(* Logix 5000 AddOnInstructionDefinition export HI1734_Faceplate_IT_AOI; software revision 30.00 *)

ADD_ON_INSTRUCTION HI1734_Faceplate_IT_AOI   (* revision 1.6, vendor Hardy Process Solutions *)
// For Integrated Technician data
VAR_IN_OUT
   Inp_hi1734 : HI:1734_WS:I:0; {required}
   Out_hi1734 : HI:1734_WS:O:0; {required}
END_VAR
VAR_INPUT
   IT_Status : DINT;   // Integrated Technician status indication
   pm_4990 : REAL;   // WT ch 0
   pm_4991 : REAL;   // Wt ch 1
   pm_4992 : REAL;   // WT ch 2
   pm_4993 : REAL;   // WT ch 3
   pm_4994 : REAL;   // WT ch 4
   pm_4995 : REAL;   // WT ch 5
   pm_4996 : REAL;   // WT ch 6
   pm_4997 : REAL;   // WT ch 7
   pm_49A0 : REAL;   // mv/v ch 0
   pm_49A1 : REAL;   // mv/v ch 1
   pm_49A2 : REAL;   // mv/v ch 2
   pm_49A3 : REAL;   // mv/v ch 3
   pm_49A8 : REAL;   // mv/v ref 1
   pm_49A4 : REAL;   // mv/v ch 4
   pm_49A5 : REAL;   // mv/v ch 5
   pm_49A6 : REAL;   // mv/v ch 6
   pm_49A7 : REAL;   // mv/v ch 7
   pm_49A9 : REAL;   // mv/v ref 2
   pm_49B0 : REAL;   // RAW VAR ch 0
   pm_49B1 : REAL;   // RAW VAR ch 1
   pm_49B2 : REAL;   // RAW VAR ch 2
   pm_49B3 : REAL;   // RAW VAR ch 3
   pm_49B8 : REAL;   // RAW VAR ref 1
   pm_49B4 : REAL;   // RAW VAR ch 4
   pm_49B5 : REAL;   // RAW VAR ch 5
   pm_49B6 : REAL;   // RAW VAR ch 6
   pm_49B7 : REAL;   // RAW VAR ch 7
   pm_49B9 : REAL;   // RAW VAR ref 2
   pm_49C0 : REAL;   // WAVERSAVER VAR ch 0
   pm_49C1 : REAL;   // WAVERSAVER VAR ch 1
   pm_49C2 : REAL;   // WAVERSAVER VAR ch 2
   pm_49C3 : REAL;   // WAVERSAVER VAR ch 3
   pm_49C8 : REAL;   // WAVERSAVER VAR ref 1
   pm_49C4 : REAL;   // WAVERSAVER VAR ch 4
   pm_49C5 : REAL;   // WAVERSAVER VAR ch 5
   pm_49C6 : REAL;   // WAVERSAVER VAR ch 6
   pm_49C7 : REAL;   // WAVERSAVER VAR ch 7
   pm_49C9 : REAL;   // WAVERSAVER VAR ref 2
   pm_49D0 : DINT;   // RAW VAR results ch 0
   pm_49D1 : DINT;   // RAW VAR results ch 1
   pm_49D2 : DINT;   // RAW VAR results ch 2
   pm_49D3 : DINT;   // RAW VAR results ch 3
   pm_49D8 : DINT;   // RAW VAR results ref 1
   pm_49D4 : DINT;   // RAW VAR results ch 4
   pm_49D5 : DINT;   // RAW VAR results ch 5
   pm_49D6 : DINT;   // RAW VAR results ch 6
   pm_49D7 : DINT;   // RAW VAR results ch 7
   pm_49D9 : DINT;   // RAW VAR results ref 2
   pm_49E0 : DINT;   // WAVERSAVER VAR results ch 0
   pm_49E1 : DINT;   // WAVERSAVER VAR results ch 1
   pm_49E2 : DINT;   // WAVERSAVER VAR results ch 2
   pm_49E3 : DINT;   // WAVERSAVER VAR results ch 3
   pm_49E8 : DINT;   // WAVERSAVER VAR results ref 1
   pm_49E4 : DINT;   // WAVERSAVER VAR results ch 4
   pm_49E5 : DINT;   // WAVERSAVER VAR results ch 5
   pm_49E6 : DINT;   // WAVERSAVER VAR results ch 6
   pm_49E7 : DINT;   // WAVERSAVER VAR results ch 7
   pm_49E9 : DINT;   // WAVERSAVER VAR results ref 2
   rd_rtz : INT;   // return to zero status
   pm_49F0 : DINT;   // RTZ ch 0
   pm_49F1 : DINT;   // RTZ ch 1
   pm_49F2 : DINT;   // RTZ ch 2
   pm_49F3 : DINT;   // RTZ ch 3
   pm_49F4 : DINT;   // RTZ ch 4
   pm_49F5 : DINT;   // RTZ ch 5
   pm_49F6 : DINT;   // RTZ ch 6
   pm_49F7 : DINT;   // RTZ ch 7
   pm_498C : DINT;   // RTZ combined
   IT_button : INT;   // IT cmd from faceplate
        .0   // IT cmd from faceplate
   pm_4881 : DINT;   // Number IT jboxes
   pm_4103 : DINT;   // Number C2 sensors
   pm_498D : DINT;   // num sensors jbox 1
   pm_498E : DINT;   // num sensors jbox 2
   IT_reduce_button : INT;   // IT reduced cmd from faceplate
        .0   // IT reduced cmd from faceplate
   IT_running_status : DINT;   // running/status indication
END_VAR
VAR
   rd_IT_wt : INT; {access None}   // Trigger to check weights
   rd_mVV : INT; {access None}   // trigger to read mv/v
   rd_raw_var : INT; {access None}   // trigger to read raw variation
   rd_ws_var : INT; {access None}   // trigger to read WAVERSAVER variation
   rd_raw_rst : INT; {access None}   // trigger to read raw variation results
   rd_ws_rst : INT; {access None}   // trigger to read WAVERSAVER results
   wr_jbox_2 : BOOL; {access None}   // Process control bit
   IT_request : INT; {access None}   // type 1=standard 2=reduced
   IT_cmd : INT;   // trigger to run IT test
   type_IT_cmd : BOOL; {access None}   // process control bit
   c2_search : BOOL; {access None}   // process control bit
   rd_C2_devices : BOOL; {access None}   // trigger to check for devices
   jbox_check : BOOL; {access None}   // j-box check process bit
   one_jbox : BOOL; {access None}   // One IT j-box found indication
   two_jbox : BOOL; {access None}   // two IT j-box indication
   run_IT_test : BOOL; {access None}   // Process control bit
   cmd_IT : DINT; {access None}   // holding register for command to be run
   IT_complete : BOOL; {access None}   // process status bit
   IT_failed : BOOL; {access None}   // process status bit
   start_timer100 : BOOL; {access None}   // process control bit
   delay100 : TIMER := (PRE := 500); {access None}   // delay to allow process to complete
   start_timer101 : BOOL; {access None}   // process control bit
   delay101 : TIMER := (PRE := 200); {access None}   // delay to allow process to complete
   start_timer102 : BOOL; {access None}   // process control bit
   delay102 : TIMER := (PRE := 200); {access None}   // delay to allow process to complete
   start_timer103 : BOOL; {access None}   // process control bit
   delay103 : TIMER := (PRE := 200); {access None}   // delay to allow process to complete
   start_timer104 : BOOL; {access None}   // process control bit
   delay104 : TIMER := (PRE := 200); {access None}   // delay to allow process to complete
   start_timer105 : BOOL; {access None}   // process control bit
   delay105 : TIMER := (PRE := 200); {access None}   // delay to allow process to complete
   start_timer106 : BOOL; {access None}   // process control bit
   delay106 : TIMER := (PRE := 200); {access None}   // delay to allow process to complete
   start_timer107 : BOOL; {access None}   // process control bit
   delay107 : TIMER := (PRE := 200); {access None}   // delay to allow process to complete
   start_timer108 : BOOL; {access None}   // process control bit
   delay108 : TIMER := (PRE := 200); {access None}   // delay to allow process to complete
   start_timer109 : BOOL; {access None}   // process control bit
   delay109 : TIMER := (PRE := 200); {access None}   // delay to allow process to complete
   start_timer110 : BOOL; {access None}   // process control bit
   delay110 : TIMER := (PRE := 200); {access None}   // delay to allow process to complete
   start_timer111 : BOOL; {access None}   // process control bit
   delay111 : TIMER := (PRE := 200); {access None}   // delay to allow process to complete
   start_timer112 : BOOL; {access None}   // process control bit
   delay112 : TIMER := (PRE := 200); {access None}   // delay to allow process to complete
   start_timer113 : BOOL; {access None}   // process control bit
   delay113 : TIMER := (PRE := 200); {access None}   // delay to allow process to complete
   start_timer114 : BOOL; {access None}   // process control bit
   delay114 : TIMER := (PRE := 200); {access None}   // delay to allow process to complete
   start_timer115 : BOOL; {access None}   // process control bit
   delay115 : TIMER := (PRE := 200); {access None}   // delay to allow process to complete
   start_timer116 : BOOL; {access None}   // process control bit
   delay116 : TIMER := (PRE := 200); {access None}   // delay to allow process to complete
   start_timer117 : BOOL; {access None}   // process control bit
   delay117 : TIMER := (PRE := 200); {access None}   // delay to allow process to complete
   start_timer118 : BOOL; {access None}   // process control bit
   start_timer119 : BOOL; {access None}   // process control bit
   delay118 : TIMER := (PRE := 200); {access None}   // delay to allow process to complete
   delay119 : TIMER := (PRE := 200); {access None}   // delay to allow process to complete
   start_timer120 : BOOL; {access None}   // process control bit
   delay120 : TIMER := (PRE := 200); {access None}   // delay to allow process to complete
   start_timer121 : BOOL; {access None}   // process control bit
   delay121 : TIMER := (PRE := 200); {access None}   // delay to allow process to complete
   start_timer122 : BOOL; {access None}   // process control bit
   delay122 : TIMER := (PRE := 200); {access None}   // delay to allow process to complete
   start_timer123 : BOOL; {access None}   // process control bit
   delay123 : TIMER := (PRE := 200); {access None}   // delay to allow process to complete
   start_timer124 : BOOL; {access None}   // process control bit
   delay124 : TIMER := (PRE := 200); {access None}   // delay to allow process to complete
   start_timer125 : BOOL; {access None}   // process control bit
   delay125 : TIMER := (PRE := 200); {access None}   // delay to allow process to complete
   start_timer126 : BOOL; {access None}   // process control bit
   delay126 : TIMER := (PRE := 200); {access None}   // delay to allow process to complete
   start_timer127 : BOOL; {access None}   // process control bit
   delay127 : TIMER := (PRE := 200); {access None}   // delay to allow process to complete
   start_timer128 : BOOL; {access None}   // process control bit
   delay128 : TIMER := (PRE := 200); {access None}   // delay to allow process to complete
   start_timer129 : BOOL; {access None}   // process control bit
   delay129 : TIMER := (PRE := 200); {access None}   // delay to allow process to complete
   start_timer130 : BOOL; {access None}   // process control bit
   delay130 : TIMER := (PRE := 200); {access None}   // delay to allow process to complete
   start_timer131 : BOOL; {access None}   // process control bit
   delay131 : TIMER := (PRE := 200); {access None}   // delay to allow process to complete
   start_timer132 : BOOL; {access None}   // process control bit
   delay132 : TIMER := (PRE := 200); {access None}   // delay to allow process to complete
   start_timer133 : BOOL; {access None}   // process control bit
   delay133 : TIMER := (PRE := 200); {access None}   // delay to allow process to complete
   start_timer134 : BOOL; {access None}   // process control bit
   writ_box1_lc_cnt : BOOL; {access None}   // Process control bit
   delay134 : TIMER := (PRE := 200); {access None}   // delay to allow process to complete
   writ_box2_lc_cnt : BOOL; {access None}   // Process control bit
   start_timer135 : BOOL; {access None}   // process control bit
   delay135 : TIMER := (PRE := 200); {access None}   // delay to allow process to complete
   run_C2_search : BOOL; {access None}   // Process control bit
   c2_dev_notmatch : BOOL; {access None}   // status indication bit
   total_sensors : DINT; {access None}   // total sensors indication
   clear_status : BOOL; {access None}   // process control bit
   delay138 : TIMER := (PRE := 5000); {access None}   // delay to allow process to complete
   start_timer139 : BOOL; {access None}   // process control bit
   delay139 : TIMER := (PRE := 200); {access None}   // delay to allow process to complete
   start_timer141 : BOOL; {access None}   // process control bit
   delay142 : TIMER := (PRE := 2000); {access None}   // delay to allow process to complete
   no_it_jbox : BOOL; {access None}   // no IT j-box indication
   rd_jbox_2_too : BOOL; {access None}   // Process control bit
END_VAR

ROUTINE Logic   (* ladder *)
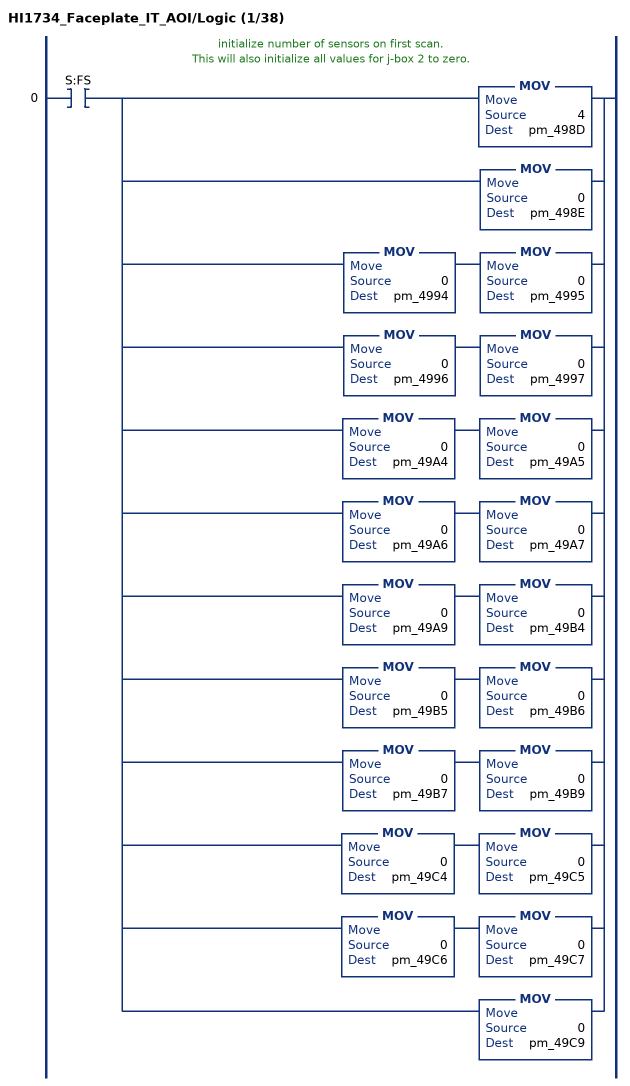
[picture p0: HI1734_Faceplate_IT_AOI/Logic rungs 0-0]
   // initialize number of sensors on first scan.
   // This will also initialize all values for j-box 2 to zero.
   0: XIC(S:FS)[MOV(4,pm_498D) ,MOV(0,pm_498E) ,MOV(0,pm_4994) MOV(0,pm_4995) ,MOV(0,pm_4996) MOV(0,pm_4997) ,MOV(0,pm_49A4) MOV(0,pm_49A5) ,MOV(0,pm_49A6) MOV(0,pm_49A7) ,MOV(0,pm_49A9) MOV(0,pm_49B4) ,MOV(0,pm_49B5) MOV(0,pm_49B6) ,MOV(0,pm_49B7) MOV(0,pm_49B9) ,MOV(0,pm_49C4) MOV(0,pm_49C5) ,MOV(0,pm_49C6) MOV(0,pm_49C7) ,MOV(0,pm_49C9) ];
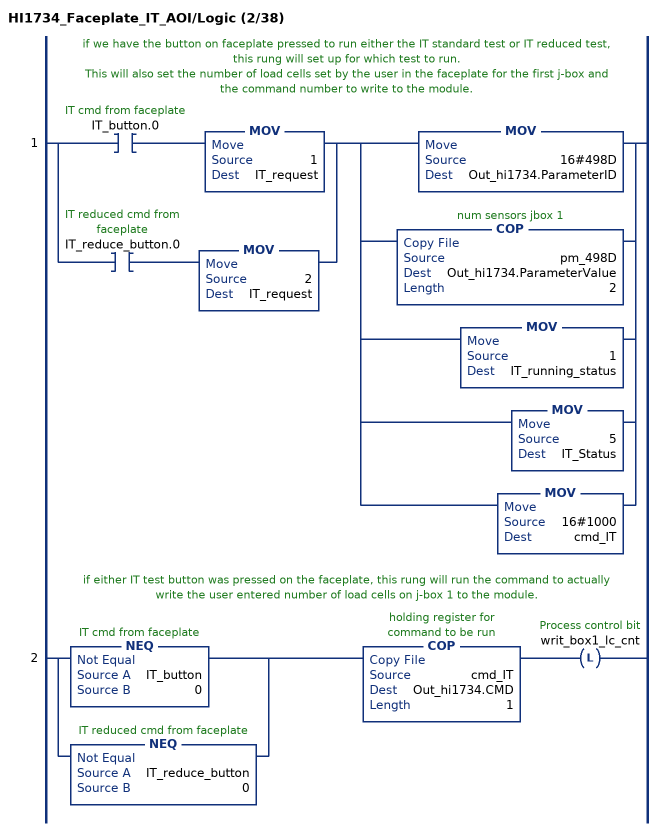
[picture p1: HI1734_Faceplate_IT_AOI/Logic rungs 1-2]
   // if we have the button on faceplate pressed to run either the IT standard test or IT reduced test, this rung will set up for which test to run.
   // This will also set the number of load cells set by the user in the faceplate for the first j-box and the command number to write to the module.
   1: [XIC(IT_button.0) MOV(1,IT_request) ,XIC(IT_reduce_button.0) MOV(2,IT_request) ][MOV(16#498D,Out_hi1734.ParameterID) ,COP(pm_498D,Out_hi1734.ParameterValue,2) ,MOV(1,IT_running_status) ,MOV(5,IT_Status) ,MOV(16#1000,cmd_IT) ];
   // if either IT test button was pressed on the faceplate, this rung will run the command to actually write the user entered number of load cells on j-box 1 to the module.
   2: [NEQ(IT_button,0) ,NEQ(IT_reduce_button,0) ]COP(cmd_IT,Out_hi1734.CMD,1)OTL(writ_box1_lc_cnt);
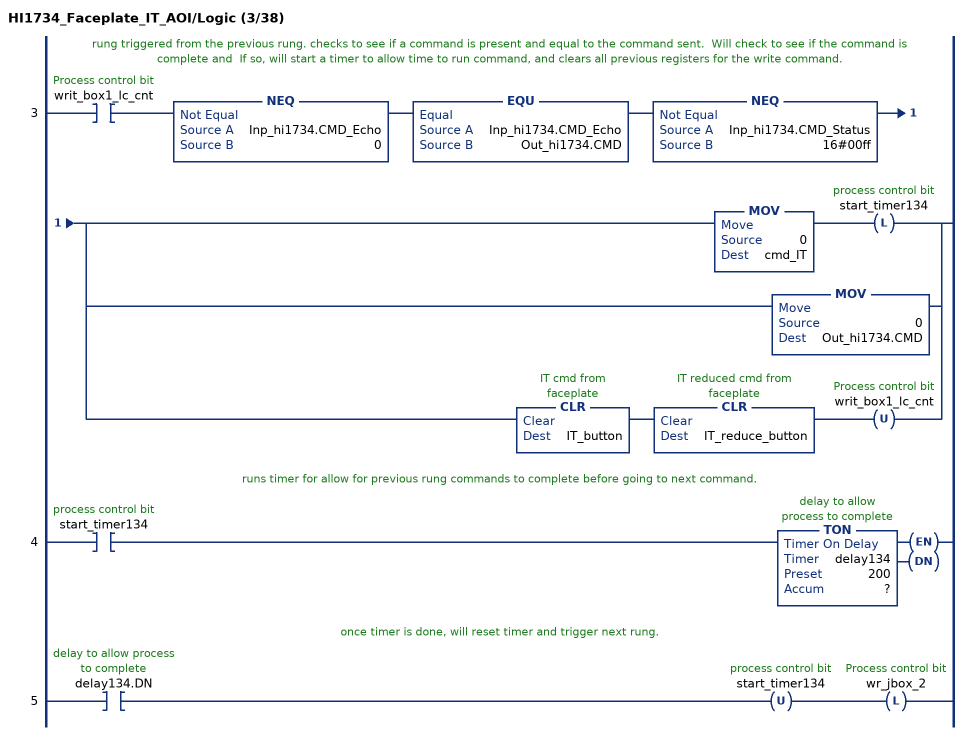
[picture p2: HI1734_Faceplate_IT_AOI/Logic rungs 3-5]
   // rung triggered from the previous rung. checks to see if a command is present and equal to the command sent.  Will check to see if the command is complete and  If so, will start a timer to allow time to run command, and clears all previous registers for the write command.
   3: XIC(writ_box1_lc_cnt)NEQ(Inp_hi1734.CMD_Echo,0)EQU(Inp_hi1734.CMD_Echo,Out_hi1734.CMD)NEQ(Inp_hi1734.CMD_Status,16#00ff)[MOV(0,cmd_IT) OTL(start_timer134) ,MOV(0,Out_hi1734.CMD) ,CLR(IT_button) CLR(IT_reduce_button) OTU(writ_box1_lc_cnt) ];
   // runs timer for allow for previous rung commands to complete before going to next command.
   4: XIC(start_timer134)TON(delay134,?,?);
   // once timer is done, will reset timer and trigger next rung.
   5: XIC(delay134.DN)OTU(start_timer134)OTL(wr_jbox_2);
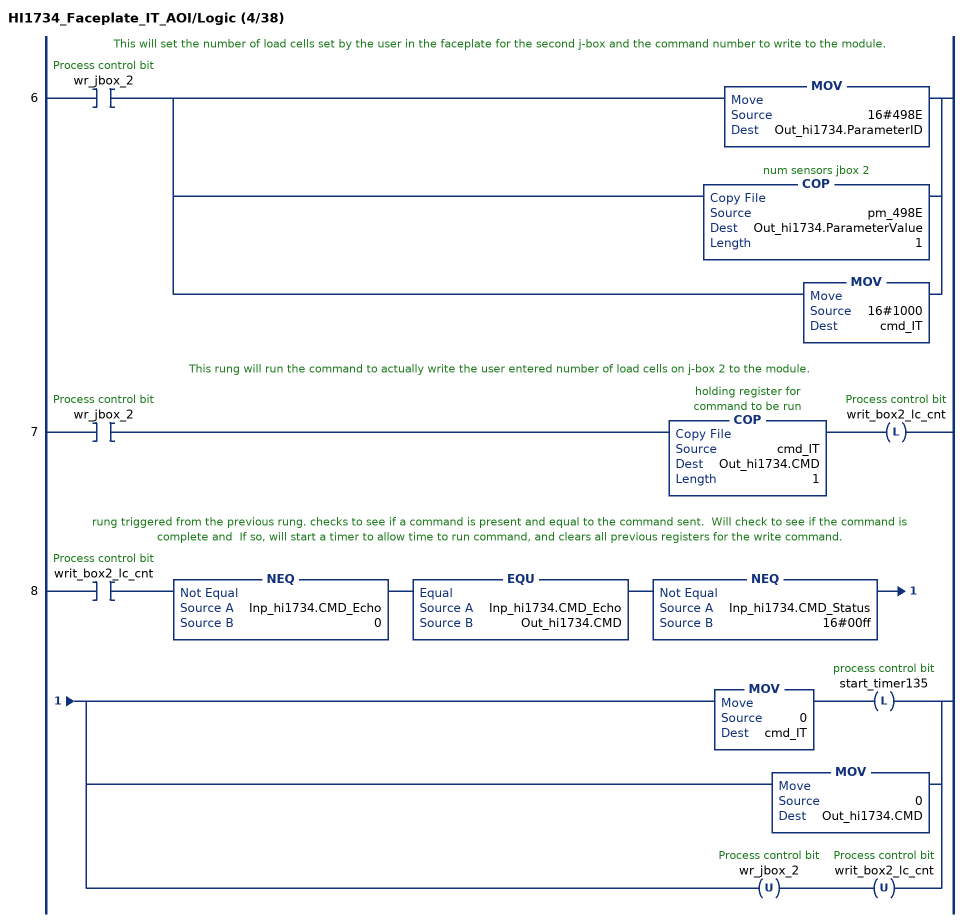
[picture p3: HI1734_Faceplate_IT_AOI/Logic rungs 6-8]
   // This will set the number of load cells set by the user in the faceplate for the second j-box and the command number to write to the module.
   6: XIC(wr_jbox_2)[MOV(16#498E,Out_hi1734.ParameterID) ,COP(pm_498E,Out_hi1734.ParameterValue,1) ,MOV(16#1000,cmd_IT) ];
   // This rung will run the command to actually write the user entered number of load cells on j-box 2 to the module.
   7: XIC(wr_jbox_2)COP(cmd_IT,Out_hi1734.CMD,1)OTL(writ_box2_lc_cnt);
   // rung triggered from the previous rung. checks to see if a command is present and equal to the command sent.  Will check to see if the command is complete and  If so, will start a timer to allow time to run command, and clears all previous registers for the write command.
   8: XIC(writ_box2_lc_cnt)NEQ(Inp_hi1734.CMD_Echo,0)EQU(Inp_hi1734.CMD_Echo,Out_hi1734.CMD)NEQ(Inp_hi1734.CMD_Status,16#00ff)[MOV(0,cmd_IT) OTL(start_timer135) ,MOV(0,Out_hi1734.CMD) ,OTU(wr_jbox_2) OTU(writ_box2_lc_cnt) ];
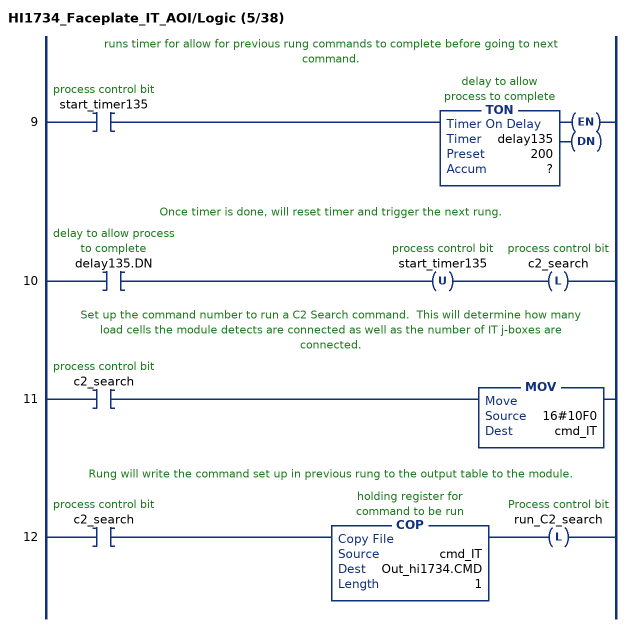
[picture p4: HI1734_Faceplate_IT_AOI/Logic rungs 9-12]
   // runs timer for allow for previous rung commands to complete before going to next command.
   9: XIC(start_timer135)TON(delay135,?,?);
   // Once timer is done, will reset timer and trigger the next rung.
   10: XIC(delay135.DN)OTU(start_timer135)OTL(c2_search);
   // Set up the command number to run a C2 Search command.  This will determine how many load cells the module detects are connected as well as the number of IT j-boxes are connected.
   11: XIC(c2_search)MOV(16#10F0,cmd_IT);
   // Rung will write the command set up in previous rung to the output table to the module.
   12: XIC(c2_search)COP(cmd_IT,Out_hi1734.CMD,1)OTL(run_C2_search);
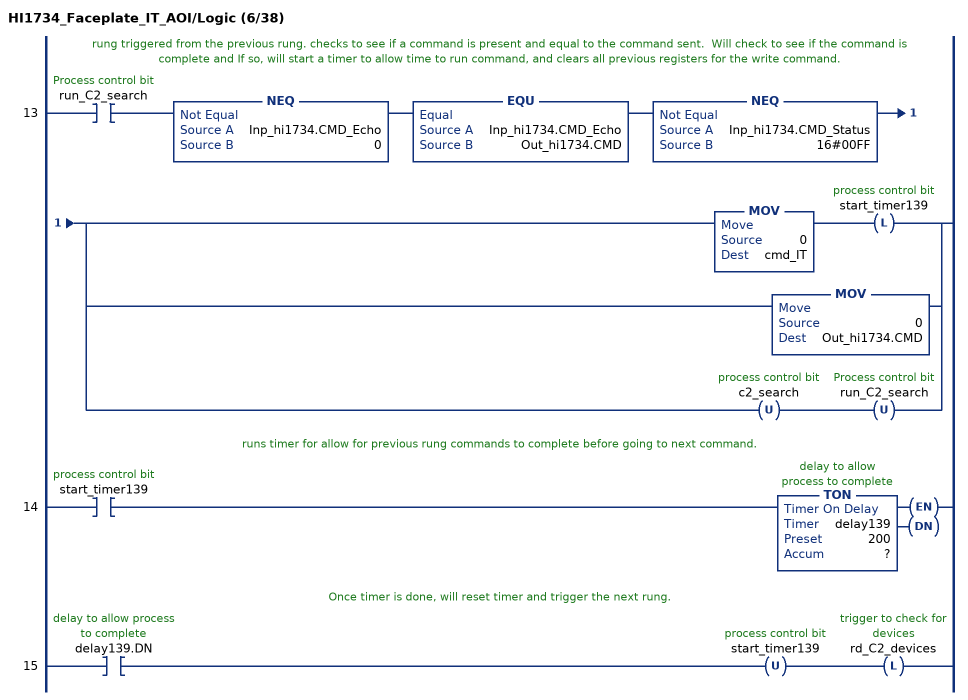
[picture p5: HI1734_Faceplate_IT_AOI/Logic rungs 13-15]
   // rung triggered from the previous rung. checks to see if a command is present and equal to the command sent.  Will check to see if the command is complete and If so, will start a timer to allow time to run command, and clears all previous registers for the write command.
   13: XIC(run_C2_search)NEQ(Inp_hi1734.CMD_Echo,0)EQU(Inp_hi1734.CMD_Echo,Out_hi1734.CMD)NEQ(Inp_hi1734.CMD_Status,16#00FF)[MOV(0,cmd_IT) OTL(start_timer139) ,MOV(0,Out_hi1734.CMD) ,OTU(c2_search) OTU(run_C2_search) ];
   // runs timer for allow for previous rung commands to complete before going to next command.
   14: XIC(start_timer139)TON(delay139,?,?);
   // Once timer is done, will reset timer and trigger the next rung.
   15: XIC(delay139.DN)OTU(start_timer139)OTL(rd_C2_devices);
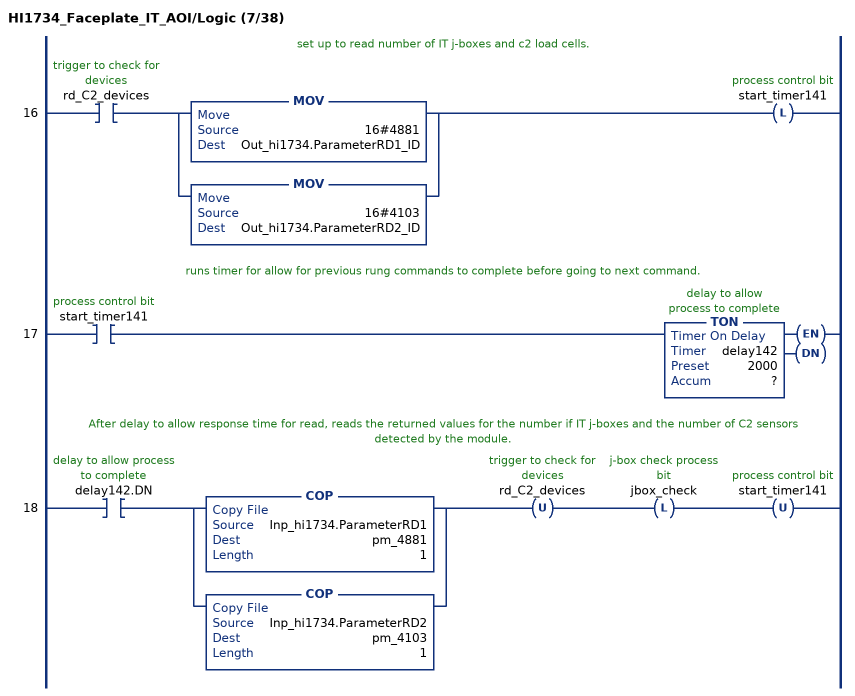
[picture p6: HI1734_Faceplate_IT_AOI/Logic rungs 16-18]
   // set up to read number of IT j-boxes and c2 load cells.
   16: XIC(rd_C2_devices)[MOV(16#4881,Out_hi1734.ParameterRD1_ID) ,MOV(16#4103,Out_hi1734.ParameterRD2_ID) ]OTL(start_timer141);
   // runs timer for allow for previous rung commands to complete before going to next command.
   17: XIC(start_timer141)TON(delay142,?,?);
   // After delay to allow response time for read, reads the returned values for the number if IT j-boxes and the number of C2 sensors detected by the module.
   18: XIC(delay142.DN)[COP(Inp_hi1734.ParameterRD1,pm_4881,1) ,COP(Inp_hi1734.ParameterRD2,pm_4103,1) ]OTU(rd_C2_devices)OTL(jbox_check)OTU(start_timer141);
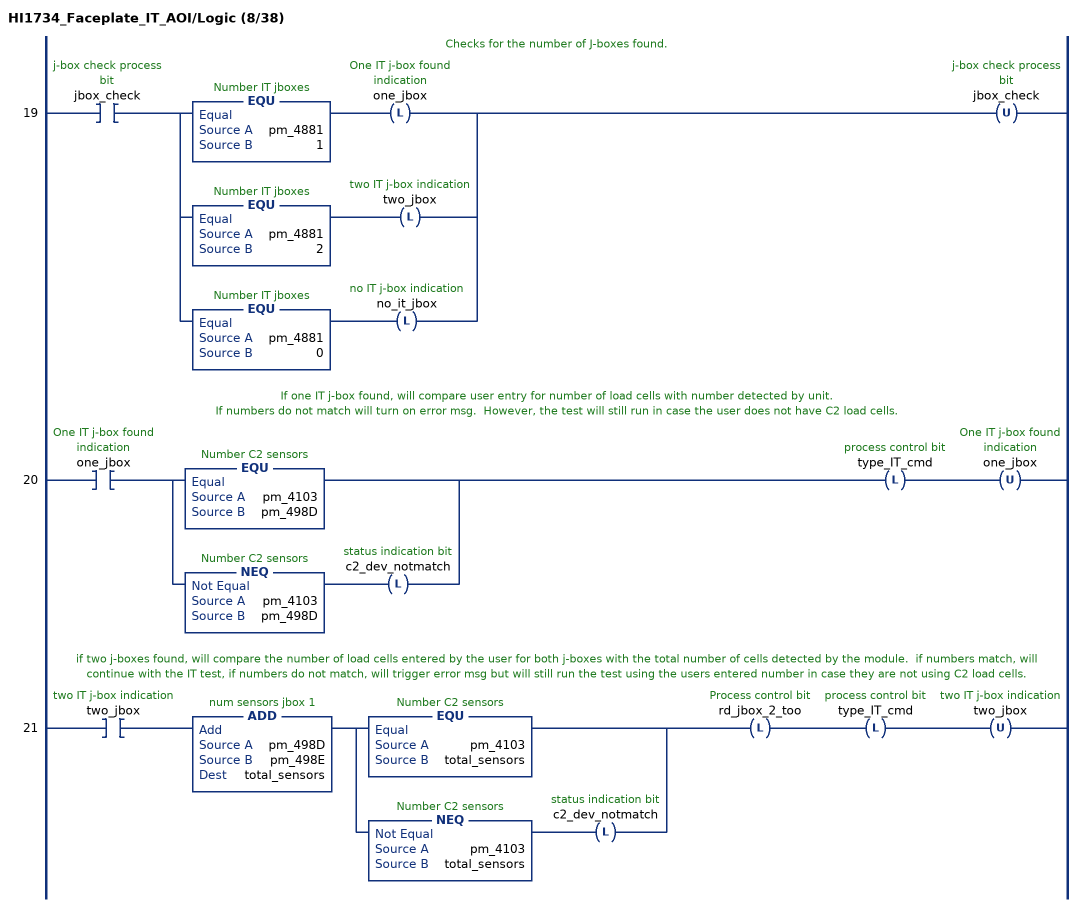
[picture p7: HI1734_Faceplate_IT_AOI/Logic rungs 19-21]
   // Checks for the number of J-boxes found.
   19: XIC(jbox_check)[EQU(pm_4881,1) OTL(one_jbox) ,EQU(pm_4881,2) OTL(two_jbox) ,EQU(pm_4881,0) OTL(no_it_jbox) ]OTU(jbox_check);
   // If one IT j-box found, will compare user entry for number of load cells with number detected by unit.
   // If numbers do not match will turn on error msg.  However, the test will still run in case the user does not have C2 load cells.
   20: XIC(one_jbox)[EQU(pm_4103,pm_498D) ,NEQ(pm_4103,pm_498D) OTL(c2_dev_notmatch) ]OTL(type_IT_cmd)OTU(one_jbox);
   // if two j-boxes found, will compare the number of load cells entered by the user for both j-boxes with the total number of cells detected by the module.  if numbers match, will continue with the IT test, if numbers do not match, will trigger error msg but will still run the test using the users entered number in case they are not using C2 load cells.
   21: XIC(two_jbox)ADD(pm_498D,pm_498E,total_sensors)[EQU(pm_4103,total_sensors) ,NEQ(pm_4103,total_sensors) OTL(c2_dev_notmatch) ]OTL(rd_jbox_2_too)OTL(type_IT_cmd)OTU(two_jbox);
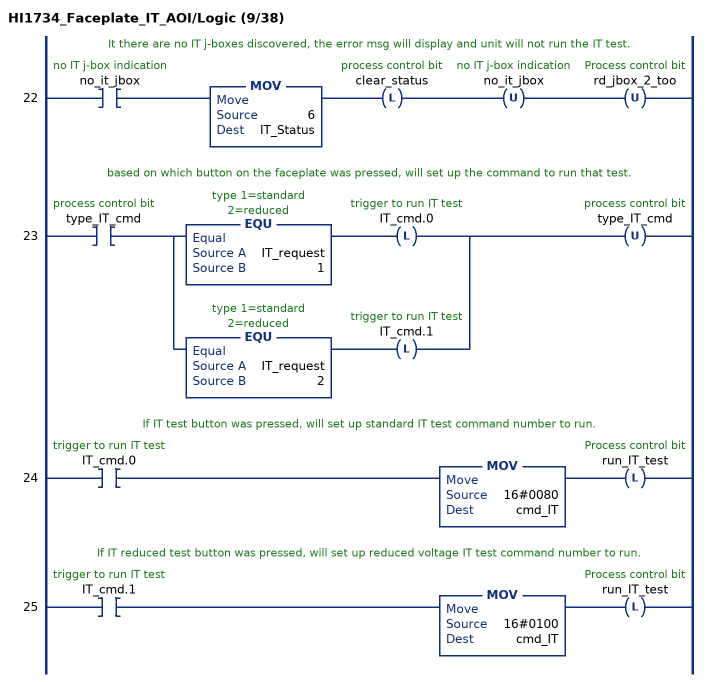
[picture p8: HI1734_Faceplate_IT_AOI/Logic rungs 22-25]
   // It there are no IT j-boxes discovered, the error msg will display and unit will not run the IT test.
   22: XIC(no_it_jbox)MOV(6,IT_Status)OTL(clear_status)OTU(no_it_jbox)OTU(rd_jbox_2_too);
   // based on which button on the faceplate was pressed, will set up the command to run that test.
   23: XIC(type_IT_cmd)[EQU(IT_request,1) OTL(IT_cmd.0) ,EQU(IT_request,2) OTL(IT_cmd.1) ]OTU(type_IT_cmd);
   // If IT test button was pressed, will set up standard IT test command number to run.
   24: XIC(IT_cmd.0)MOV(16#0080,cmd_IT)OTL(run_IT_test);
   // If IT reduced test button was pressed, will set up reduced voltage IT test command number to run.
   25: XIC(IT_cmd.1)MOV(16#0100,cmd_IT)OTL(run_IT_test);
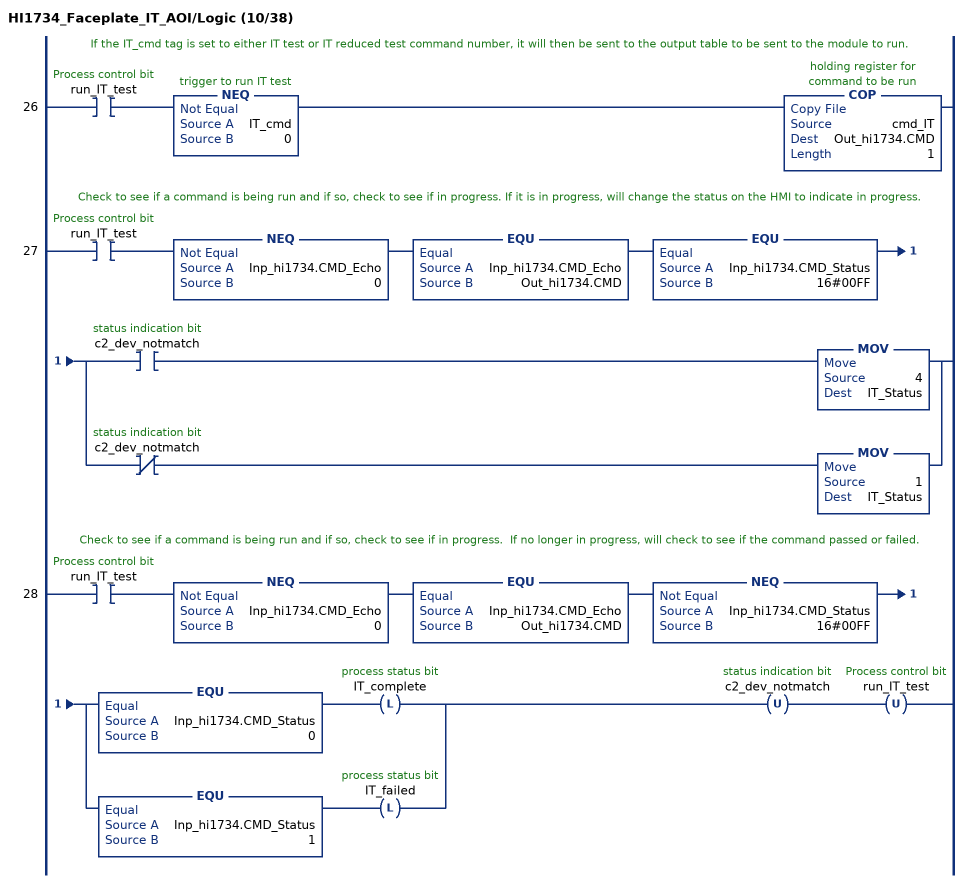
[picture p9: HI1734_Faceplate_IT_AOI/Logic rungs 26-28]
   // If the IT_cmd tag is set to either IT test or IT reduced test command number, it will then be sent to the output table to be sent to the module to run.
   26: XIC(run_IT_test)NEQ(IT_cmd,0)COP(cmd_IT,Out_hi1734.CMD,1);
   // Check to see if a command is being run and if so, check to see if in progress. If it is in progress, will change the status on the HMI to indicate in progress.
   27: XIC(run_IT_test)NEQ(Inp_hi1734.CMD_Echo,0)EQU(Inp_hi1734.CMD_Echo,Out_hi1734.CMD)EQU(Inp_hi1734.CMD_Status,16#00FF)[XIC(c2_dev_notmatch) MOV(4,IT_Status) ,XIO(c2_dev_notmatch) MOV(1,IT_Status) ];
   // Check to see if a command is being run and if so, check to see if in progress.  If no longer in progress, will check to see if the command passed or failed.
   28: XIC(run_IT_test)NEQ(Inp_hi1734.CMD_Echo,0)EQU(Inp_hi1734.CMD_Echo,Out_hi1734.CMD)NEQ(Inp_hi1734.CMD_Status,16#00FF)[EQU(Inp_hi1734.CMD_Status,0) OTL(IT_complete) ,EQU(Inp_hi1734.CMD_Status,1) OTL(IT_failed) ]OTU(c2_dev_notmatch)OTU(run_IT_test);
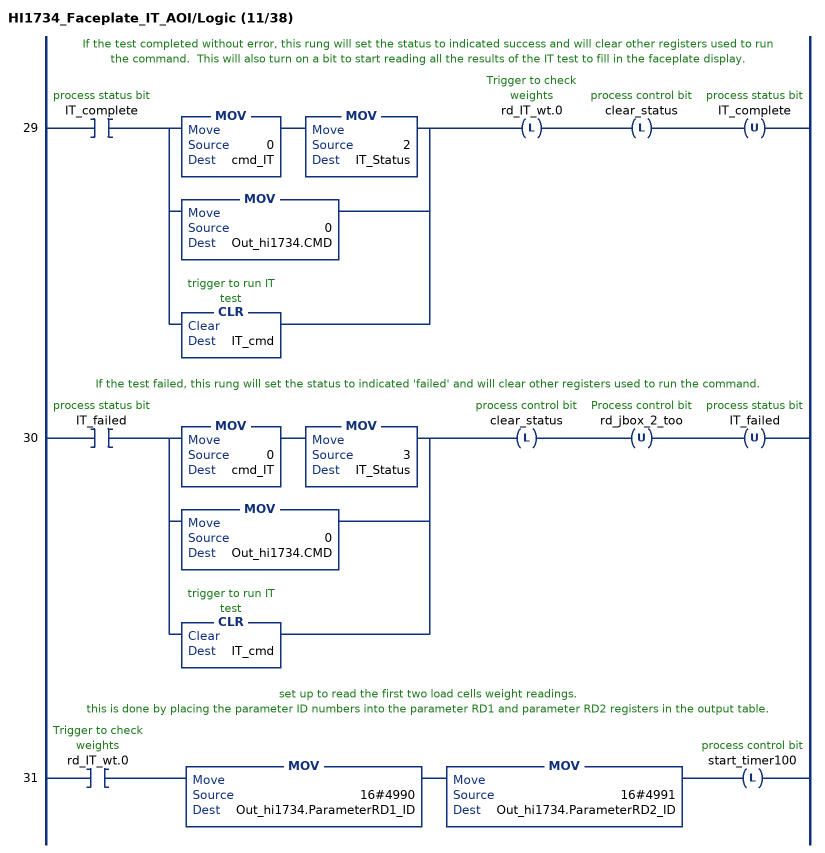
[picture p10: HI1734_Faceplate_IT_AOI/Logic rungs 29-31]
   // If the test completed without error, this rung will set the status to indicated success and will clear other registers used to run the command.  This will also turn on a bit to start reading all the results of the IT test to fill in the faceplate display.
   29: XIC(IT_complete)[MOV(0,cmd_IT) MOV(2,IT_Status) ,MOV(0,Out_hi1734.CMD) ,CLR(IT_cmd) ]OTL(rd_IT_wt.0)OTL(clear_status)OTU(IT_complete);
   // If the test failed, this rung will set the status to indicated 'failed' and will clear other registers used to run the command.
   30: XIC(IT_failed)[MOV(0,cmd_IT) MOV(3,IT_Status) ,MOV(0,Out_hi1734.CMD) ,CLR(IT_cmd) ]OTL(clear_status)OTU(rd_jbox_2_too)OTU(IT_failed);
   // set up to read the first two load cells weight readings.
   // this is done by placing the parameter ID numbers into the parameter RD1 and parameter RD2 registers in the output table.
   31: XIC(rd_IT_wt.0)MOV(16#4990,Out_hi1734.ParameterRD1_ID)MOV(16#4991,Out_hi1734.ParameterRD2_ID)OTL(start_timer100);
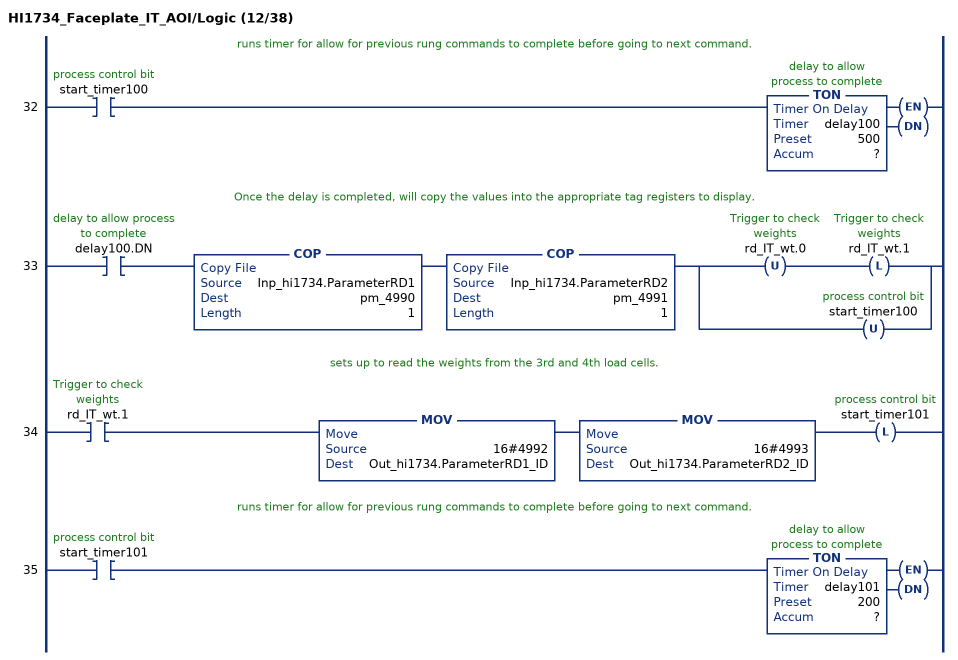
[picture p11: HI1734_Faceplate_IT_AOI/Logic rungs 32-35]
   // runs timer for allow for previous rung commands to complete before going to next command.
   32: XIC(start_timer100)TON(delay100,?,?);
   // Once the delay is completed, will copy the values into the appropriate tag registers to display.
   33: XIC(delay100.DN)COP(Inp_hi1734.ParameterRD1,pm_4990,1)COP(Inp_hi1734.ParameterRD2,pm_4991,1)[OTU(rd_IT_wt.0) OTL(rd_IT_wt.1) ,OTU(start_timer100) ];
   // sets up to read the weights from the 3rd and 4th load cells.
   34: XIC(rd_IT_wt.1)MOV(16#4992,Out_hi1734.ParameterRD1_ID)MOV(16#4993,Out_hi1734.ParameterRD2_ID)OTL(start_timer101);
   // runs timer for allow for previous rung commands to complete before going to next command.
   35: XIC(start_timer101)TON(delay101,?,?);
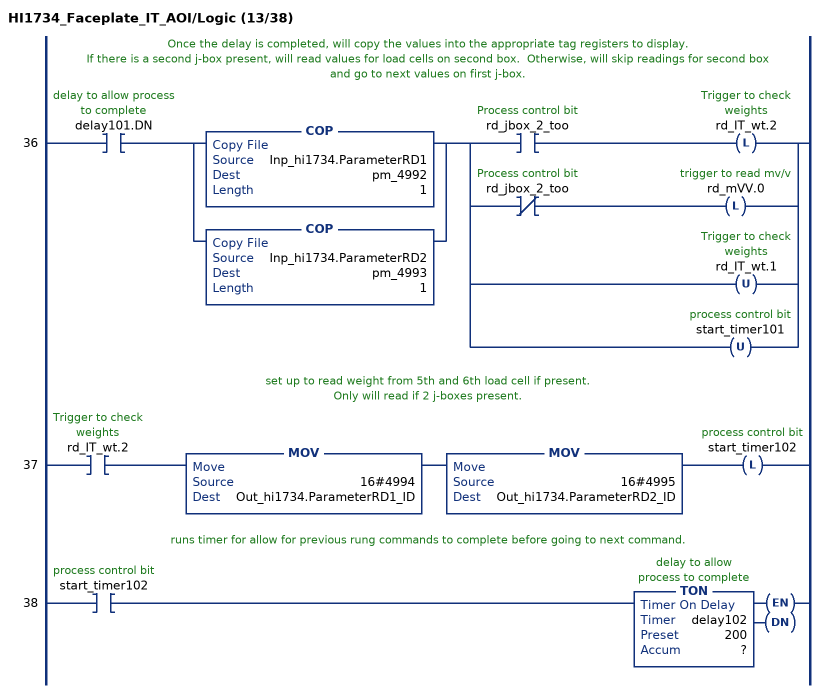
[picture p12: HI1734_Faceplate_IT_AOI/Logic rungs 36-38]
   // Once the delay is completed, will copy the values into the appropriate tag registers to display.
   // If there is a second j-box present, will read values for load cells on second box.  Otherwise, will skip readings for second box and go to next values on first j-box.
   36: XIC(delay101.DN)[COP(Inp_hi1734.ParameterRD1,pm_4992,1) ,COP(Inp_hi1734.ParameterRD2,pm_4993,1) ][XIC(rd_jbox_2_too) OTL(rd_IT_wt.2) ,XIO(rd_jbox_2_too) OTL(rd_mVV.0) ,OTU(rd_IT_wt.1) ,OTU(start_timer101) ];
   // set up to read weight from 5th and 6th load cell if present.
   // Only will read if 2 j-boxes present.
   37: XIC(rd_IT_wt.2)MOV(16#4994,Out_hi1734.ParameterRD1_ID)MOV(16#4995,Out_hi1734.ParameterRD2_ID)OTL(start_timer102);
   // runs timer for allow for previous rung commands to complete before going to next command.
   38: XIC(start_timer102)TON(delay102,?,?);
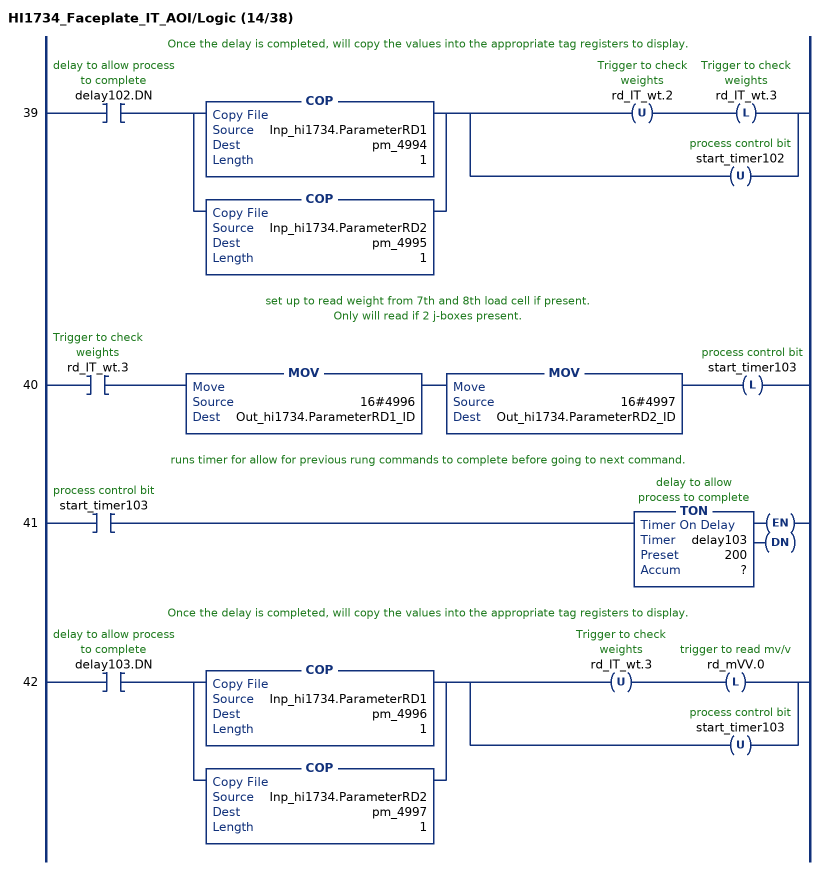
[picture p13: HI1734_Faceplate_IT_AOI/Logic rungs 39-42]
   // Once the delay is completed, will copy the values into the appropriate tag registers to display.
   39: XIC(delay102.DN)[COP(Inp_hi1734.ParameterRD1,pm_4994,1) ,COP(Inp_hi1734.ParameterRD2,pm_4995,1) ][OTU(rd_IT_wt.2) OTL(rd_IT_wt.3) ,OTU(start_timer102) ];
   // set up to read weight from 7th and 8th load cell if present.
   // Only will read if 2 j-boxes present.
   40: XIC(rd_IT_wt.3)MOV(16#4996,Out_hi1734.ParameterRD1_ID)MOV(16#4997,Out_hi1734.ParameterRD2_ID)OTL(start_timer103);
   // runs timer for allow for previous rung commands to complete before going to next command.
   41: XIC(start_timer103)TON(delay103,?,?);
   // Once the delay is completed, will copy the values into the appropriate tag registers to display.
   42: XIC(delay103.DN)[COP(Inp_hi1734.ParameterRD1,pm_4996,1) ,COP(Inp_hi1734.ParameterRD2,pm_4997,1) ][OTU(rd_IT_wt.3) OTL(rd_mVV.0) ,OTU(start_timer103) ];
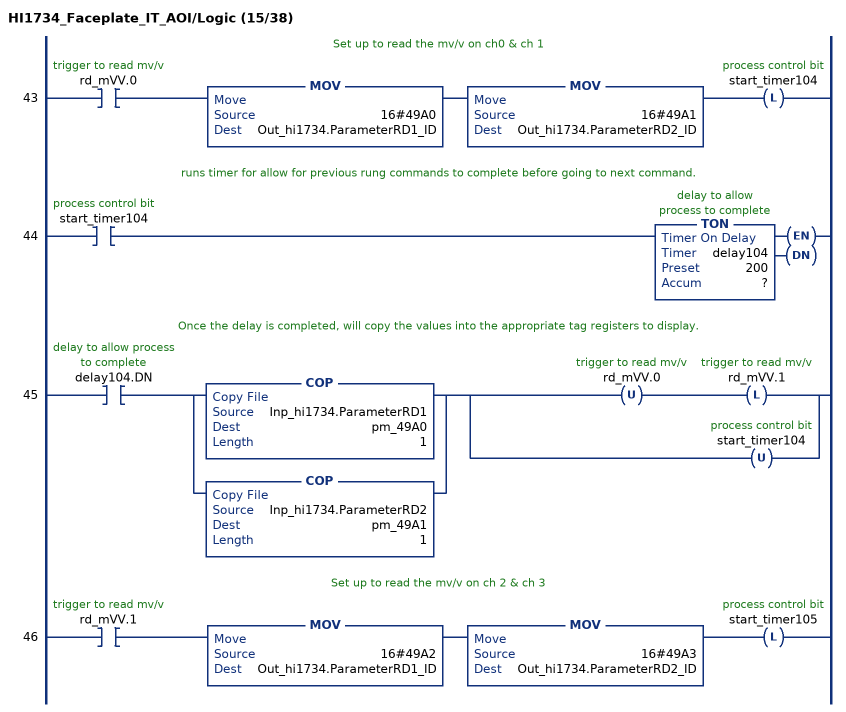
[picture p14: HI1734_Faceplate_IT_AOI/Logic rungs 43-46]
   // Set up to read the mv/v on ch0 & ch 1
   43: XIC(rd_mVV.0)MOV(16#49A0,Out_hi1734.ParameterRD1_ID)MOV(16#49A1,Out_hi1734.ParameterRD2_ID)OTL(start_timer104);
   // runs timer for allow for previous rung commands to complete before going to next command.
   44: XIC(start_timer104)TON(delay104,?,?);
   // Once the delay is completed, will copy the values into the appropriate tag registers to display.
   45: XIC(delay104.DN)[COP(Inp_hi1734.ParameterRD1,pm_49A0,1) ,COP(Inp_hi1734.ParameterRD2,pm_49A1,1) ][OTU(rd_mVV.0) OTL(rd_mVV.1) ,OTU(start_timer104) ];
   // Set up to read the mv/v on ch 2 & ch 3
   46: XIC(rd_mVV.1)MOV(16#49A2,Out_hi1734.ParameterRD1_ID)MOV(16#49A3,Out_hi1734.ParameterRD2_ID)OTL(start_timer105);
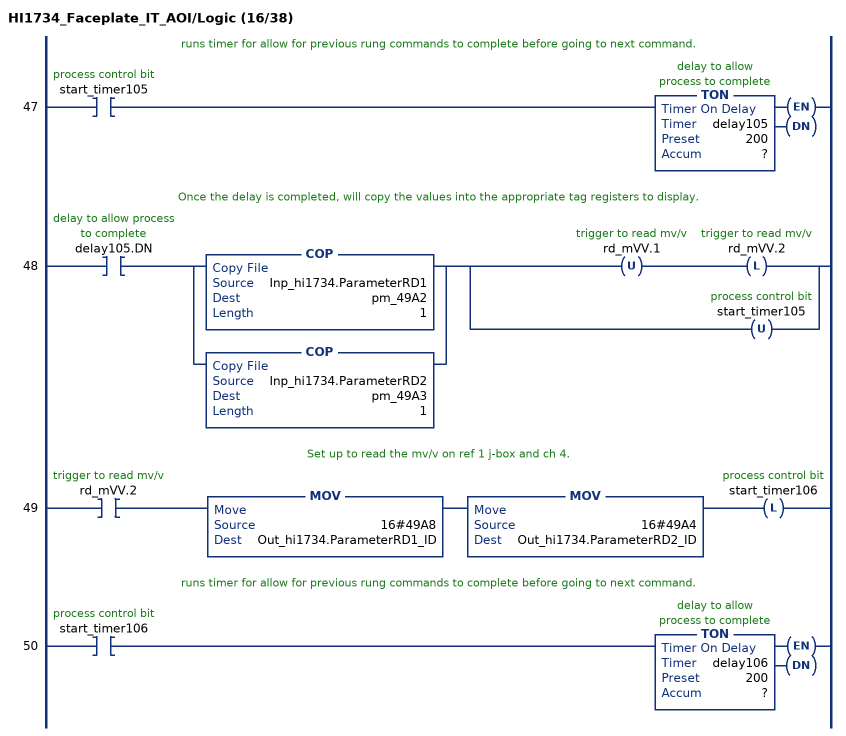
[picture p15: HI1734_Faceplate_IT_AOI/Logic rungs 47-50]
   // runs timer for allow for previous rung commands to complete before going to next command.
   47: XIC(start_timer105)TON(delay105,?,?);
   // Once the delay is completed, will copy the values into the appropriate tag registers to display.
   48: XIC(delay105.DN)[COP(Inp_hi1734.ParameterRD1,pm_49A2,1) ,COP(Inp_hi1734.ParameterRD2,pm_49A3,1) ][OTU(rd_mVV.1) OTL(rd_mVV.2) ,OTU(start_timer105) ];
   // Set up to read the mv/v on ref 1 j-box and ch 4.
   49: XIC(rd_mVV.2)MOV(16#49A8,Out_hi1734.ParameterRD1_ID)MOV(16#49A4,Out_hi1734.ParameterRD2_ID)OTL(start_timer106);
   // runs timer for allow for previous rung commands to complete before going to next command.
   50: XIC(start_timer106)TON(delay106,?,?);
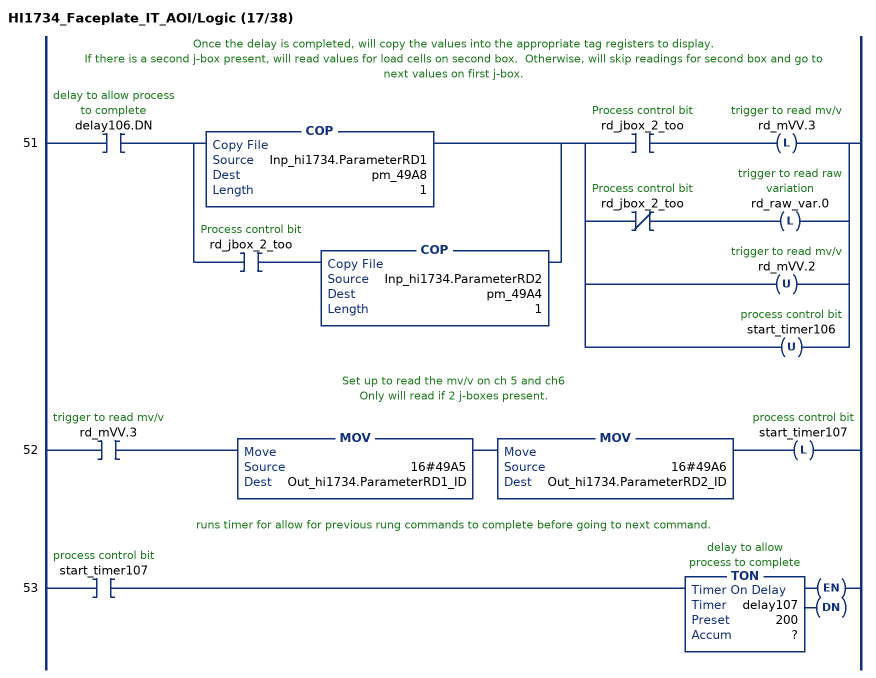
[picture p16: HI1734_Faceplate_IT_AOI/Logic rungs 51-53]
   // Once the delay is completed, will copy the values into the appropriate tag registers to display.
   // If there is a second j-box present, will read values for load cells on second box.  Otherwise, will skip readings for second box and go to next values on first j-box.
   51: XIC(delay106.DN)[COP(Inp_hi1734.ParameterRD1,pm_49A8,1) ,XIC(rd_jbox_2_too) COP(Inp_hi1734.ParameterRD2,pm_49A4,1) ][XIC(rd_jbox_2_too) OTL(rd_mVV.3) ,XIO(rd_jbox_2_too) OTL(rd_raw_var.0) ,OTU(rd_mVV.2) ,OTU(start_timer106) ];
   // Set up to read the mv/v on ch 5 and ch6
   // Only will read if 2 j-boxes present.
   52: XIC(rd_mVV.3)MOV(16#49A5,Out_hi1734.ParameterRD1_ID)MOV(16#49A6,Out_hi1734.ParameterRD2_ID)OTL(start_timer107);
   // runs timer for allow for previous rung commands to complete before going to next command.
   53: XIC(start_timer107)TON(delay107,?,?);
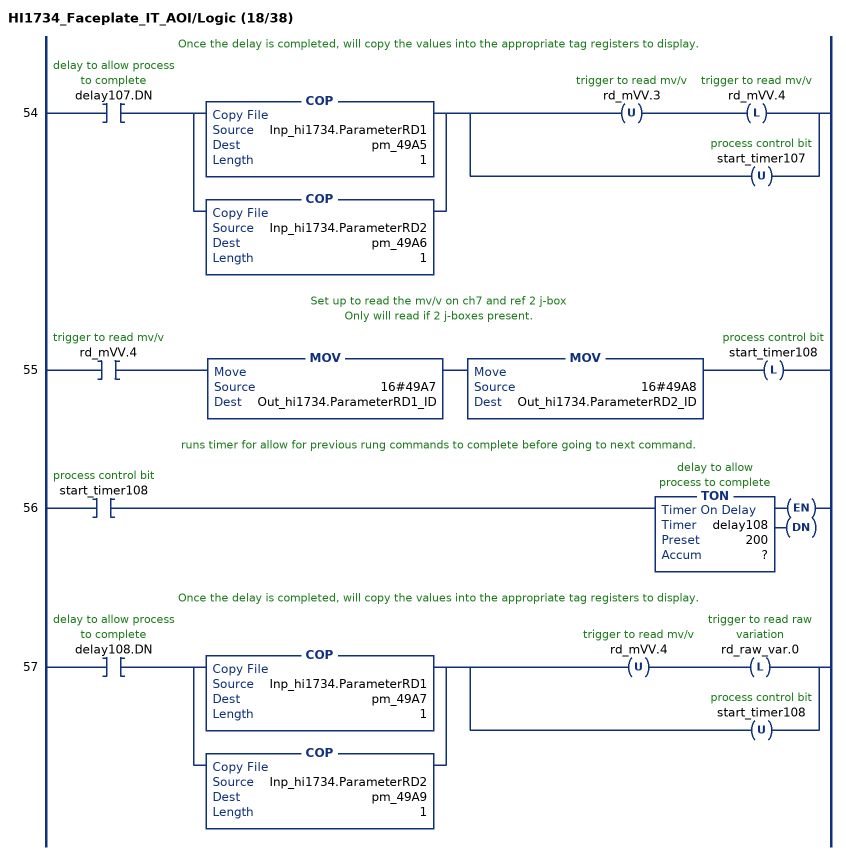
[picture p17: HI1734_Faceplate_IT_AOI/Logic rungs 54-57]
   // Once the delay is completed, will copy the values into the appropriate tag registers to display.
   54: XIC(delay107.DN)[COP(Inp_hi1734.ParameterRD1,pm_49A5,1) ,COP(Inp_hi1734.ParameterRD2,pm_49A6,1) ][OTU(rd_mVV.3) OTL(rd_mVV.4) ,OTU(start_timer107) ];
   // Set up to read the mv/v on ch7 and ref 2 j-box
   // Only will read if 2 j-boxes present.
   55: XIC(rd_mVV.4)MOV(16#49A7,Out_hi1734.ParameterRD1_ID)MOV(16#49A8,Out_hi1734.ParameterRD2_ID)OTL(start_timer108);
   // runs timer for allow for previous rung commands to complete before going to next command.
   56: XIC(start_timer108)TON(delay108,?,?);
   // Once the delay is completed, will copy the values into the appropriate tag registers to display.
   57: XIC(delay108.DN)[COP(Inp_hi1734.ParameterRD1,pm_49A7,1) ,COP(Inp_hi1734.ParameterRD2,pm_49A9,1) ][OTU(rd_mVV.4) OTL(rd_raw_var.0) ,OTU(start_timer108) ];
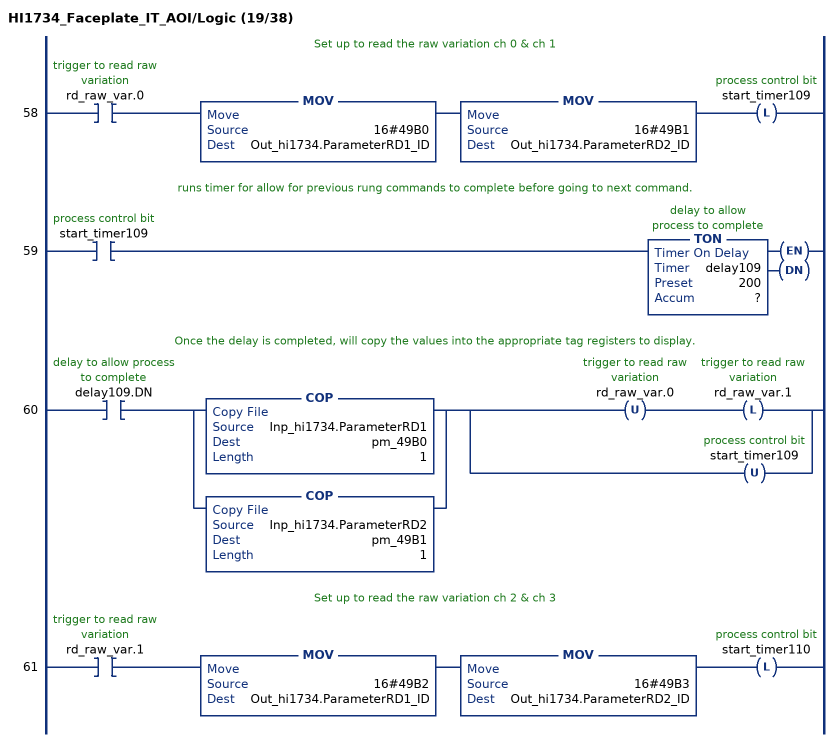
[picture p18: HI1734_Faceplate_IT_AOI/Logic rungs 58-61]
   // Set up to read the raw variation ch 0 & ch 1
   58: XIC(rd_raw_var.0)MOV(16#49B0,Out_hi1734.ParameterRD1_ID)MOV(16#49B1,Out_hi1734.ParameterRD2_ID)OTL(start_timer109);
   // runs timer for allow for previous rung commands to complete before going to next command.
   59: XIC(start_timer109)TON(delay109,?,?);
   // Once the delay is completed, will copy the values into the appropriate tag registers to display.
   60: XIC(delay109.DN)[COP(Inp_hi1734.ParameterRD1,pm_49B0,1) ,COP(Inp_hi1734.ParameterRD2,pm_49B1,1) ][OTU(rd_raw_var.0) OTL(rd_raw_var.1) ,OTU(start_timer109) ];
   // Set up to read the raw variation ch 2 & ch 3
   61: XIC(rd_raw_var.1)MOV(16#49B2,Out_hi1734.ParameterRD1_ID)MOV(16#49B3,Out_hi1734.ParameterRD2_ID)OTL(start_timer110);
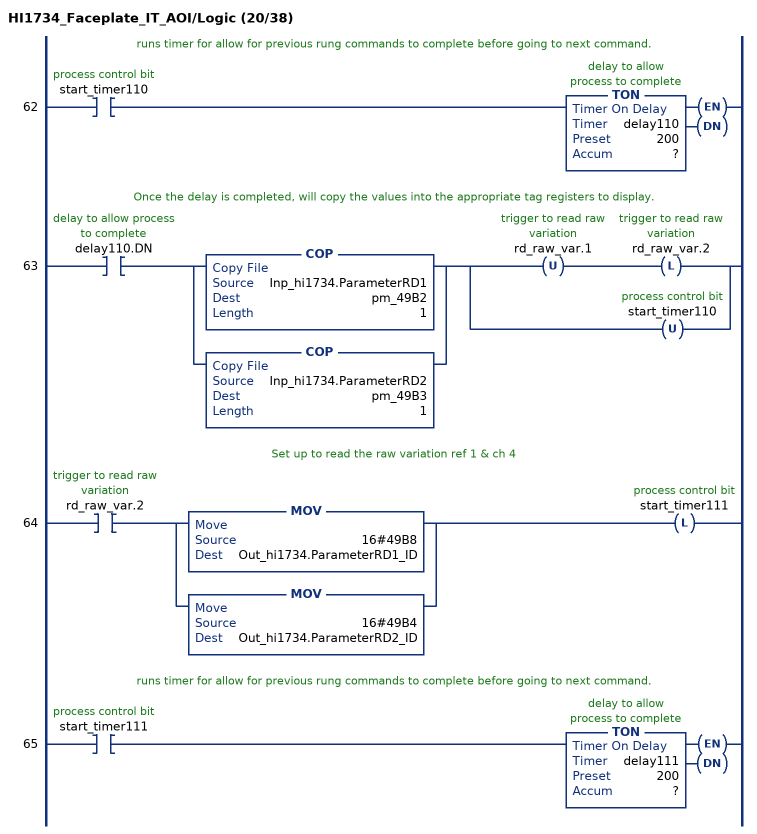
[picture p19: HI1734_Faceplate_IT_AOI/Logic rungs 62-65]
   // runs timer for allow for previous rung commands to complete before going to next command.
   62: XIC(start_timer110)TON(delay110,?,?);
   // Once the delay is completed, will copy the values into the appropriate tag registers to display.
   63: XIC(delay110.DN)[COP(Inp_hi1734.ParameterRD1,pm_49B2,1) ,COP(Inp_hi1734.ParameterRD2,pm_49B3,1) ][OTU(rd_raw_var.1) OTL(rd_raw_var.2) ,OTU(start_timer110) ];
   // Set up to read the raw variation ref 1 & ch 4
   64: XIC(rd_raw_var.2)[MOV(16#49B8,Out_hi1734.ParameterRD1_ID) ,MOV(16#49B4,Out_hi1734.ParameterRD2_ID) ]OTL(start_timer111);
   // runs timer for allow for previous rung commands to complete before going to next command.
   65: XIC(start_timer111)TON(delay111,?,?);
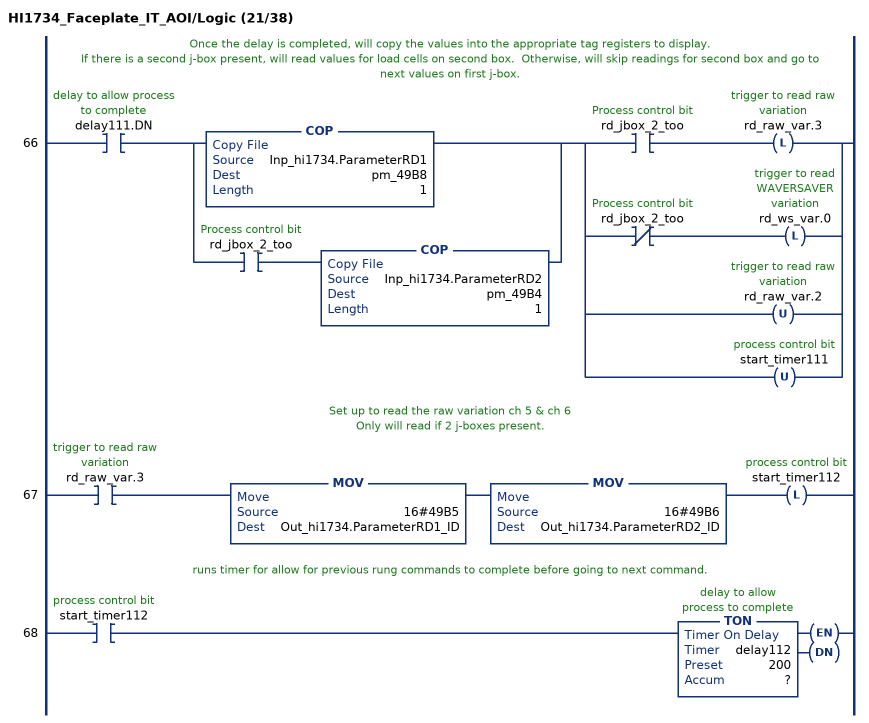
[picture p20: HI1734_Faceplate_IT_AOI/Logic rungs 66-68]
   // Once the delay is completed, will copy the values into the appropriate tag registers to display.
   // If there is a second j-box present, will read values for load cells on second box.  Otherwise, will skip readings for second box and go to next values on first j-box.
   66: XIC(delay111.DN)[COP(Inp_hi1734.ParameterRD1,pm_49B8,1) ,XIC(rd_jbox_2_too) COP(Inp_hi1734.ParameterRD2,pm_49B4,1) ][XIC(rd_jbox_2_too) OTL(rd_raw_var.3) ,XIO(rd_jbox_2_too) OTL(rd_ws_var.0) ,OTU(rd_raw_var.2) ,OTU(start_timer111) ];
   // Set up to read the raw variation ch 5 & ch 6
   // Only will read if 2 j-boxes present.
   67: XIC(rd_raw_var.3)MOV(16#49B5,Out_hi1734.ParameterRD1_ID)MOV(16#49B6,Out_hi1734.ParameterRD2_ID)OTL(start_timer112);
   // runs timer for allow for previous rung commands to complete before going to next command.
   68: XIC(start_timer112)TON(delay112,?,?);
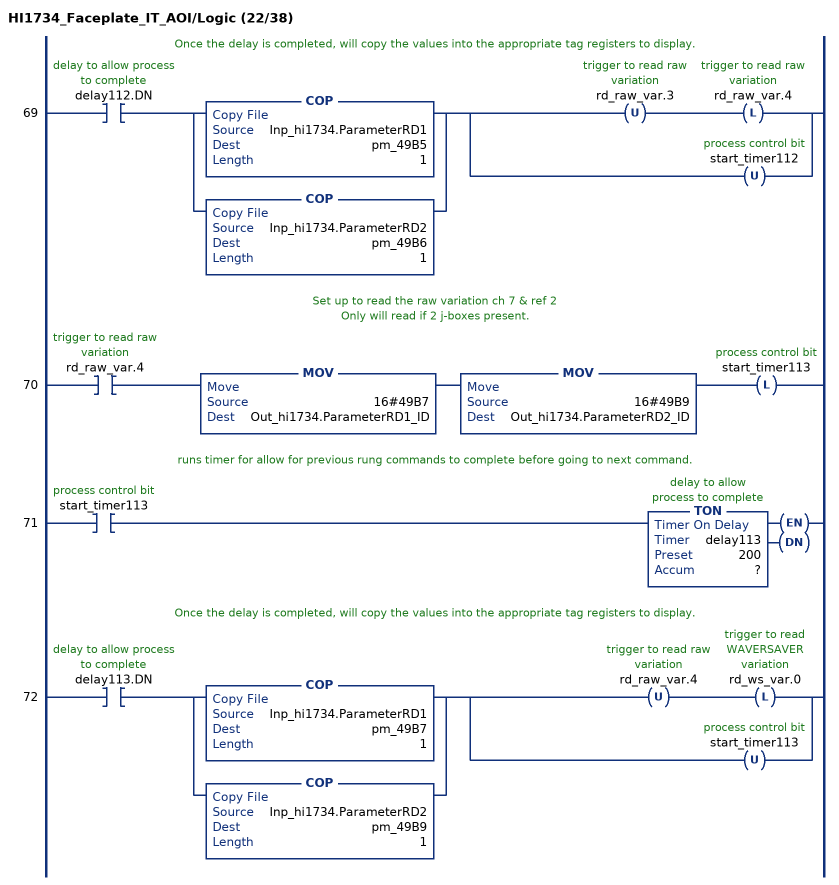
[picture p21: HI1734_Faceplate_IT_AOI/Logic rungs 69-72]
   // Once the delay is completed, will copy the values into the appropriate tag registers to display.
   69: XIC(delay112.DN)[COP(Inp_hi1734.ParameterRD1,pm_49B5,1) ,COP(Inp_hi1734.ParameterRD2,pm_49B6,1) ][OTU(rd_raw_var.3) OTL(rd_raw_var.4) ,OTU(start_timer112) ];
   // Set up to read the raw variation ch 7 & ref 2
   // Only will read if 2 j-boxes present.
   70: XIC(rd_raw_var.4)MOV(16#49B7,Out_hi1734.ParameterRD1_ID)MOV(16#49B9,Out_hi1734.ParameterRD2_ID)OTL(start_timer113);
   // runs timer for allow for previous rung commands to complete before going to next command.
   71: XIC(start_timer113)TON(delay113,?,?);
   // Once the delay is completed, will copy the values into the appropriate tag registers to display.
   72: XIC(delay113.DN)[COP(Inp_hi1734.ParameterRD1,pm_49B7,1) ,COP(Inp_hi1734.ParameterRD2,pm_49B9,1) ][OTU(rd_raw_var.4) OTL(rd_ws_var.0) ,OTU(start_timer113) ];
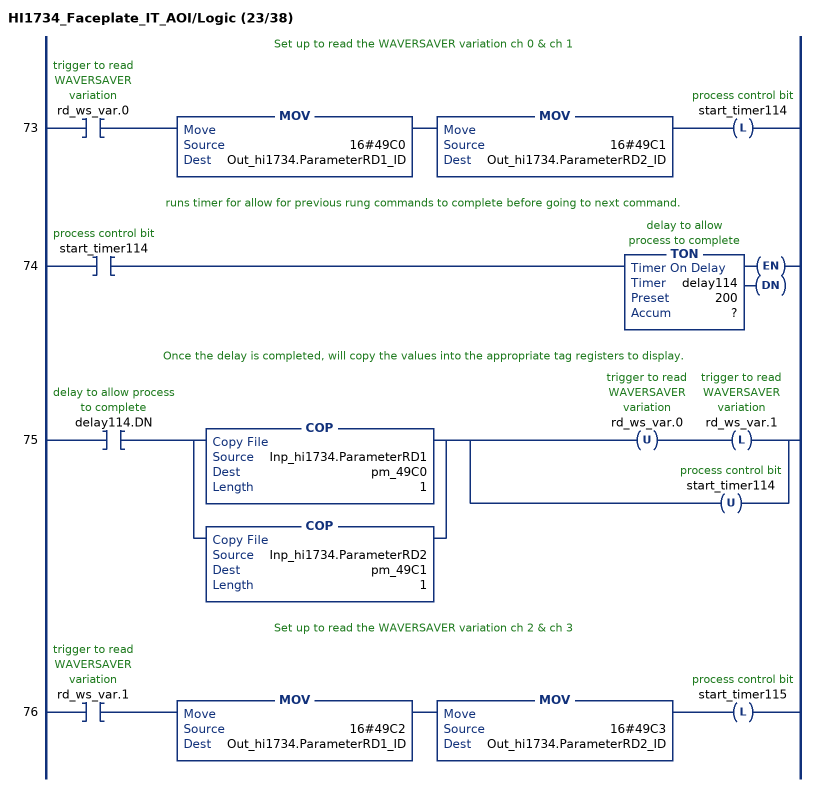
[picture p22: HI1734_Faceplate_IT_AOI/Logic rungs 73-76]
   // Set up to read the WAVERSAVER variation ch 0 & ch 1
   73: XIC(rd_ws_var.0)MOV(16#49C0,Out_hi1734.ParameterRD1_ID)MOV(16#49C1,Out_hi1734.ParameterRD2_ID)OTL(start_timer114);
   // runs timer for allow for previous rung commands to complete before going to next command.
   74: XIC(start_timer114)TON(delay114,?,?);
   // Once the delay is completed, will copy the values into the appropriate tag registers to display.
   75: XIC(delay114.DN)[COP(Inp_hi1734.ParameterRD1,pm_49C0,1) ,COP(Inp_hi1734.ParameterRD2,pm_49C1,1) ][OTU(rd_ws_var.0) OTL(rd_ws_var.1) ,OTU(start_timer114) ];
   // Set up to read the WAVERSAVER variation ch 2 & ch 3
   76: XIC(rd_ws_var.1)MOV(16#49C2,Out_hi1734.ParameterRD1_ID)MOV(16#49C3,Out_hi1734.ParameterRD2_ID)OTL(start_timer115);
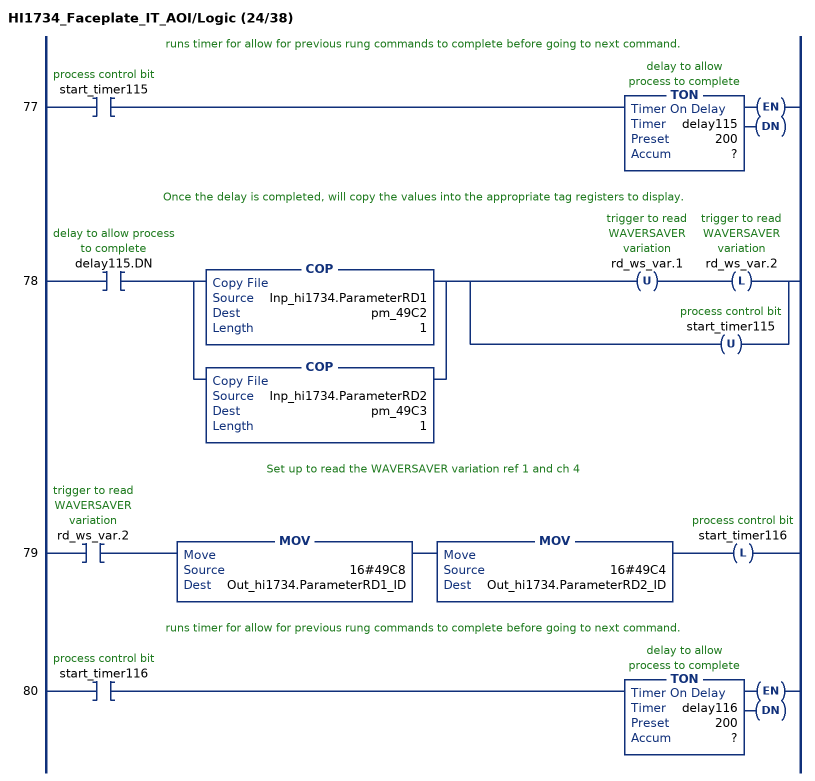
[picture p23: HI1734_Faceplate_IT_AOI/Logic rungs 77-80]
   // runs timer for allow for previous rung commands to complete before going to next command.
   77: XIC(start_timer115)TON(delay115,?,?);
   // Once the delay is completed, will copy the values into the appropriate tag registers to display.
   78: XIC(delay115.DN)[COP(Inp_hi1734.ParameterRD1,pm_49C2,1) ,COP(Inp_hi1734.ParameterRD2,pm_49C3,1) ][OTU(rd_ws_var.1) OTL(rd_ws_var.2) ,OTU(start_timer115) ];
   // Set up to read the WAVERSAVER variation ref 1 and ch 4
   79: XIC(rd_ws_var.2)MOV(16#49C8,Out_hi1734.ParameterRD1_ID)MOV(16#49C4,Out_hi1734.ParameterRD2_ID)OTL(start_timer116);
   // runs timer for allow for previous rung commands to complete before going to next command.
   80: XIC(start_timer116)TON(delay116,?,?);
